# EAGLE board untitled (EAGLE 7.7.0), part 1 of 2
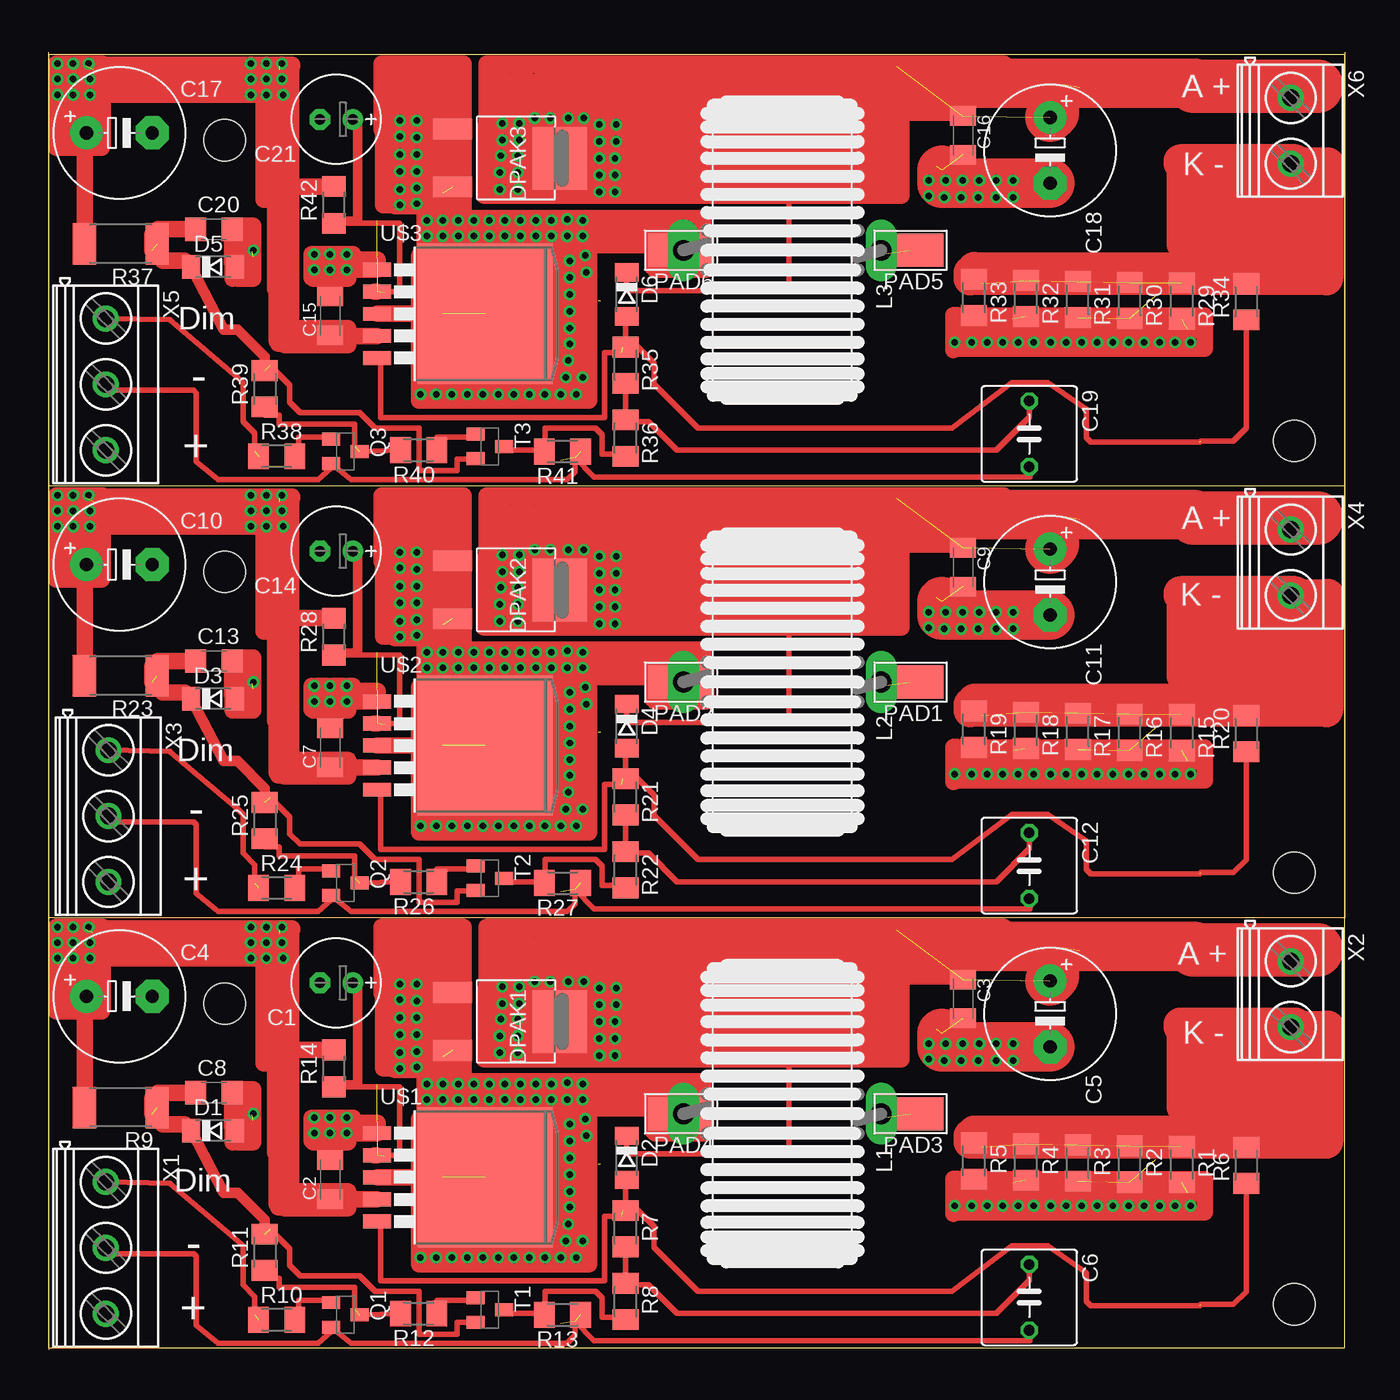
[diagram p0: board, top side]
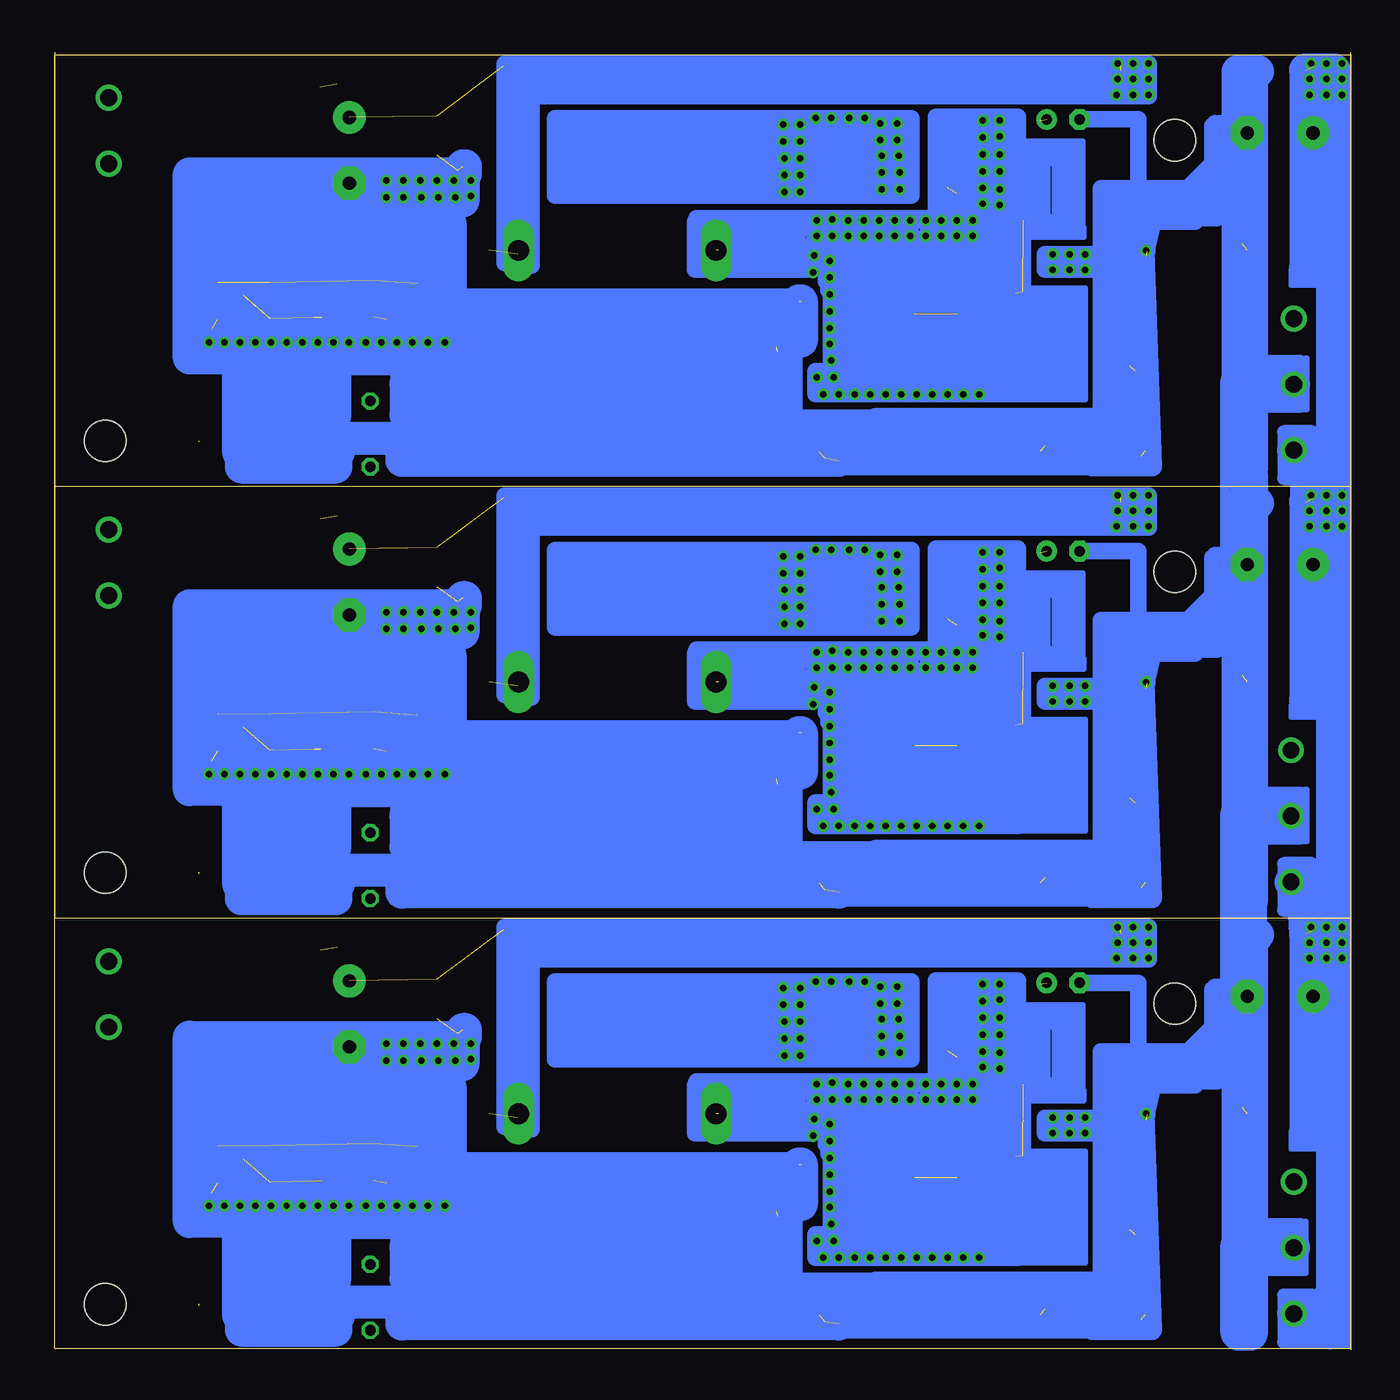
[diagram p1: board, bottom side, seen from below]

Size 100 x 100.1 mm. Coordinates in mm from the lower left corner, seen from the top.
Outline: 0,100.1 0,0.1 100,0.1 100,33.3
Outline: 100,100.1 100,33.3
Outline: 0,33.3 0,0
Outline: 100,33.3 0,33.3
Outline: 100,33.4 100,66.6 0,66.6
Outline: 0,66.6 0,33.3
Outline: 100,66.7 100,99.9 0,99.9 0,66.6
Copper layers (1*16): Top 0.035mm / dielectric 1.5mm / Bottom 0.035mm
Design rules "default": minimum track width 10mil, minimum drill 24mil, track to track 8mil, track to pad 8mil, pad to pad 8mil, via to via 8mil, smd to smd 8mil, copper to edge 40mil, drill to drill 8mil, minimum pad ring 10mil, minimum via ring 8mil, stop-mask expansion 4mil, vias tented up to drill 0mil, thermal gap 10mil
Holes 3.2 mm at 96.1,3.5 13.6,26.7 96.1,36.8 13.6,60 96.1,70.1 13.6,93.3

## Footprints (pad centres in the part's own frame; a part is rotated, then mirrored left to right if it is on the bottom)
E2,5-7 = drill 0.813 pad 1.6: + -1.27,0 | drill 0.813 pad 1.6 octagon: - 1.27,0
C1206K = smd 1.5 x 2: 1 -1.5,0; 2 1.5,0
E5-10,5 = drill 1.016 pad 2.54: + -2.54,0 | drill 1.016 pad 2.54 octagon: - 2.54,0
C050-075X075 = drill 0.813 octagon: 1 -2.54,0; 2 2.54,0
C1206 = smd 1.6 x 1.8: 1 -1.4,0; 2 1.4,0
SOD80C = smd 1.4 x 1.8: A 1.7,0; C -1.7,0
DPAK = smd 1.6 x 2.997: 1 -2.261,-4.928; 3 2.21,-4.928 | smd 4.826 x 4.191: 4 0,3.353
SFT1240 = drill 1.6 long: 1 -7.62,0; 2 7.62,0
5-2,5 = smd 2.54 x 5.08: 1 0,0
SOT23-BEC = smd 1 x 1.4: B -0.95,-1.1; C 0,1.1; E 0.95,-1.1
M1206 = smd 1.6 x 2: 1 -1.4,0; 2 1.4,0
R2512 = smd 1.8 x 3.2: 1 -2.8,0; 2 2.8,0
R1206 = smd 1.6 x 1.803: 1 -1.422,0; 2 1.422,0
TO263-5 = smd 1.067 x 2.159: 1 -3.404,-7.061; 2 -1.702,-7.061; 3 0,-7.061; 4 1.702,-7.061; 5 3.404,-7.061 | smd 10.8 x 10.41: 6 0,1.27
MKDSN1,5/3-5,08 = drill 1.3 pad 2: 1 -7.641,0.025; 2 -2.561,0.025; 3 2.519,0.025
MKDSN1,5/2-5,08 = drill 1.3 pad 2: 1 -2.561,0.025; 2 2.519,0.025

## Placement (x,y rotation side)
C1  47µ  [E2,5-7]  22.2,28.3 180 top
C2  1µ  [C1206K]  21.74,13.13 90 top
C3  1µ  [C1206K]  70.54,27.06 270 top
C4  220µ  [E5-10,5]  5.47,27.26 0 top
C5  100µ 63V  [E5-10,5]  77.26,25.91 270 top
C6  1µ  [C050-075X075]  75.65,4.04 270 top
C7  1µ  [C1206K]  21.74,46.43 90 top
C8  100n  [C1206]  12.76,19.82 0 top
C9  1µ  [C1206K]  70.54,60.36 270 top
C10  220µ  [E5-10,5]  5.47,60.56 0 top
C11  100µ 63V  [E5-10,5]  77.26,59.21 270 top
C12  1µ  [C050-075X075]  75.65,37.34 270 top
C13  100n  [C1206]  12.76,53.12 0 top
C14  47µ  [E2,5-7]  22.2,61.6 180 top
C15  1µ  [C1206K]  21.74,79.73 90 top
C16  1µ  [C1206K]  70.54,93.66 270 top
C17  220µ  [E5-10,5]  5.47,93.86 0 top
C18  100µ 63V  [E5-10,5]  77.26,92.51 270 top
C19  1µ  [C050-075X075]  75.65,70.64 270 top
C20  100n  [C1206]  12.76,86.42 0 top
C21  47µ  [E2,5-7]  22.2,94.9 180 top
D1  5,1V  [SOD80C]  12.71,16.91 0 top
D2  56V  [SOD80C]  44.6,14.8 270 top
D3  5,1V  [SOD80C]  12.71,50.21 0 top
D4  56V  [SOD80C]  44.6,48.1 270 top
D5  5,1V  [SOD80C]  12.71,83.51 0 top
D6  56V  [SOD80C]  44.6,81.4 270 top
DPAK1  1N581D  [DPAK]  36.1,25.3 270 top
DPAK2  1N581D  [DPAK]  36.1,58.6 270 top
DPAK3  1N581D  [DPAK]  36.1,91.9 270 top
L1  SFT1240  [SFT1240]  56.6,18.2 180 top
L2  SFT1240  [SFT1240]  56.6,51.5 180 top
L3  SFT1240  [SFT1240]  56.6,84.8 180 top
PAD1  WIREPADSMD5-2,5  [5-2,5]  66.5,51.5 90 top
PAD2  WIREPADSMD5-2,5  [5-2,5]  48.8,51.5 90 top
PAD3  WIREPADSMD5-2,5  [5-2,5]  66.5,18.2 90 top
PAD4  WIREPADSMD5-2,5  [5-2,5]  48.8,18.2 90 top
PAD5  WIREPADSMD5-2,5  [5-2,5]  66.5,84.8 90 top
PAD6  WIREPADSMD5-2,5  [5-2,5]  48.8,84.8 90 top
Q1  BC817  [SOT23-BEC]  22.9,2.69 270 top
Q2  BC817  [SOT23-BEC]  22.9,35.99 270 top
Q3  BC817  [SOT23-BEC]  22.9,69.29 270 top
R1  0,22  [M1206]  87.42,14.29 270 top
R2  [M1206]  83.39,14.32 270 top
R3  [M1206]  79.39,14.4 270 top
R4  [M1206]  75.39,14.48 270 top
R5  [M1206]  71.39,14.56 270 top
R6  1K  [M1206]  92.38,14.23 90 top
R7  20K  [M1206]  44.51,9.34 270 top
R8  1K  [M1206]  44.51,3.72 270 top
R9  680  [R2512]  5.58,18.69 180 top
R10  33K  [M1206]  17.6,2.31 0 top
R11  1K  [M1206]  16.69,7.52 90 top
R12  10K  [M1206]  28.56,2.79 180 top
R13  1K  [M1206]  39.64,2.69 180 top
R14  33K  [R1206]  22,21.7 90 top
R15  0,22  [M1206]  87.42,47.59 270 top
R16  [M1206]  83.39,47.62 270 top
R17  [M1206]  79.39,47.7 270 top
R18  [M1206]  75.39,47.78 270 top
R19  [M1206]  71.39,47.86 270 top
R20  1K  [M1206]  92.38,47.53 90 top
R21  20K  [M1206]  44.51,42.64 270 top
R22  1K  [M1206]  44.51,37.02 270 top
R23  680  [R2512]  5.58,51.99 180 top
R24  33K  [M1206]  17.6,35.61 0 top
R25  1K  [M1206]  16.69,40.82 90 top
R26  10K  [M1206]  28.56,36.09 180 top
R27  1K  [M1206]  39.64,35.99 180 top
R28  33K  [R1206]  22,55 90 top
R29  0,22  [M1206]  87.42,80.89 270 top
R30  [M1206]  83.39,80.92 270 top
R31  [M1206]  79.39,81 270 top
R32  [M1206]  75.39,81.08 270 top
R33  [M1206]  71.39,81.16 270 top
R34  1K  [M1206]  92.38,80.83 90 top
R35  20K  [M1206]  44.51,75.94 270 top
R36  1K  [M1206]  44.51,70.32 270 top
R37  680  [R2512]  5.58,85.29 180 top
R38  33K  [M1206]  17.6,68.91 0 top
R39  1K  [M1206]  16.69,74.12 90 top
R40  10K  [M1206]  28.56,69.39 180 top
R41  1K  [M1206]  39.64,69.29 180 top
R42  33K  [R1206]  22,88.3 90 top
T1  BC807  [SOT23-BEC]  34.04,3.07 270 top
T2  BC807  [SOT23-BEC]  34.04,36.37 270 top
T3  BC807  [SOT23-BEC]  34.04,69.67 270 top
U$1  [TO263-5]  32.4,13.3 270 top
U$2  [TO263-5]  32.4,46.6 270 top
U$3  [TO263-5]  32.4,79.9 270 top
X1  [MKDSN1,5/3-5,08]  4.4,5.3 270 top
X2  [MKDSN1,5/2-5,08]  95.8,27.4 270 top
X3  [MKDSN1,5/3-5,08]  4.6,38.6 270 top
X4  [MKDSN1,5/2-5,08]  95.8,60.7 270 top
X5  [MKDSN1,5/3-5,08]  4.4,71.9 270 top
X6  [MKDSN1,5/2-5,08]  95.8,94 270 top

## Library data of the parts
C1 C4-C6 C8 C10-C14 C17-C21 R1-R8 R10-R22 R24-R36 R38-R42 = rcl
C2 C3 C7 C9 C15 C16 R9 R23 R37 = resistor
D1-D6 = diode
DPAK1-DPAK3 = DPAK_Schottky
L1-L3 = inductors
PAD1-PAD6 = wirepad
Q1-Q3 = transistor-npn
T1-T3 = transistor
U$1-U$3 = XL6006
X1-X6 = con-phoenix-508

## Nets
+5V: C8.1 D1.C R9.1 R11.2 T1.E
+5V1: C13.1 D3.C R23.1 R25.2 T2.E
+5V2: C20.1 D5.C R37.1 R39.2 T3.E
N$1: C1.- C2.2 C3.2 C4.- C5.- C6.2 C8.2 D1.A Q1.E R1.2 R2.2 R3.2 R4.2 R5.2 R13.1 U$1.1 X1.2
N$2: DPAK1.1 DPAK1.3 L1.2 PAD4.1 U$1.3 U$1.6
N$3: C2.1 C4.+ L1.1 PAD3.1 R9.2 R14.2 U$1.4 X1.3
N$4: R1.1 R2.1 R3.1 R4.1 R5.1 R6.2 X2.2
N$5: C6.1 R7.2 R8.1
N$6: D2.A R6.1 R7.1 U$1.5
N$7: C3.1 C5.+ D2.C DPAK1.4
N$8: Q1.C R11.1 R12.2
N$9: R12.1 T1.B
N$13: R8.2 R13.2 T1.C
N$14: Q1.B R10.2
N$15: R10.1 X1.1
N$16: C7.1 C10.+ L2.1 PAD1.1 R23.2 R28.2 U$2.4 X3.3
N$17: R15.1 R16.1 R17.1 R18.1 R19.1 R20.2 X4.2
N$19: C12.1 R21.2 R22.1
N$20: Q2.C R25.1 R26.2
N$21: R22.2 R27.2 T2.C
N$22: R24.1 X3.1
N$23: Q2.B R24.2
N$24: R26.1 T2.B
N$134: C1.+ R14.1 U$1.2
N$187: DPAK2.1 DPAK2.3 L2.2 PAD2.1 U$2.3 U$2.6
N$188: C14.+ R28.1 U$2.2
N$189: C9.1 C11.+ D4.C DPAK2.4 X4.1
N$190: D4.A R20.1 R21.1 U$2.5
N$191: C7.2 C9.2 C11.- C12.2 C13.2 C14.- D3.A Q2.E R15.2 R16.2 R17.2 R18.2 R19.2 R27.1 U$2.1 X3.2
N$291: C15.1 C17.+ L3.1 PAD5.1 R37.2 R42.2 U$3.4 X5.3
N$292: R29.1 R30.1 R31.1 R32.1 R33.1 R34.2 X6.2
N$293: C19.1 R35.2 R36.1
N$294: Q3.C R39.1 R40.2
N$295: R36.2 R41.2 T3.C
N$296: R38.1 X5.1
N$297: Q3.B R38.2
N$298: R40.1 T3.B
N$332: DPAK3.1 DPAK3.3 L3.2 PAD6.1 U$3.3 U$3.6
N$333: C21.+ R42.1 U$3.2
N$334: C16.1 C18.+ D6.C DPAK3.4
N$335: D6.A R34.1 R35.1 U$3.5
N$336: C15.2 C16.2 C17.- C18.- C19.2 C20.2 C21.- D5.A Q3.E R29.2 R30.2 R31.2 R32.2 R33.2 R41.1 U$3.1 X5.2
S$8: C10.-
